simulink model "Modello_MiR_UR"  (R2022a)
settings: Solver=FixedStepAuto  StartTime=0.0  StopTime=time_s(end,1)  FixedStep=Sim.dt*10  RelTol=1e-3  EnableMultiTasking=on
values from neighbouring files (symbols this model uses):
  a = 0.250    (= 0.25)    [Modello_MiR_UR_script.m]    (also in Modello_MiR_2ruote_script.m; Modello_MiR_6ruote_script.m; Modello_MiR_6ruote_validato_script.m)
  a1 = 0.18265    [Modello_MiR_UR_script.m]    (also in UR_DHtable_e.m = 0; Modello_MiR_2ruote_script.m = deg2rad(5); Modello_MiR_6ruote_script.m = deg2rad(5); Modello_MiR_6ruote_validato_script.m)
  a2 = 0.40857    [Modello_MiR_UR_script.m]    (also in UR_DHtable_e.m = 612; Modello_MiR_2ruote_script.m = deg2rad(25); Modello_MiR_6ruote_script.m = deg2rad(25); Modello_MiR_6ruote_validato_script.m)
  Att_C1 = 0.01    [Modello_MiR_UR_script.m]    (also in Modello_MiR_6ruote_validato_script.m)
  Att_C2 = 0.01    [Modello_MiR_UR_script.m]    (also in Modello_MiR_6ruote_validato_script.m)
  Att_C5 = 0.01    [Modello_MiR_UR_script.m]    (also in Modello_MiR_6ruote_validato_script.m)
  Att_C6 = 0.01    [Modello_MiR_UR_script.m]    (also in Modello_MiR_6ruote_validato_script.m)
  b = 0.1875    [Modello_MiR_UR_script.m]    (also in Modello_MiR_2ruote_script.m; Modello_MiR_6ruote_script.m; Modello_MiR_6ruote_validato_script.m)
  b_caster = 0.07    [Modello_MiR_UR_script.m]    (also in Modello_MiR_2ruote_script.m; Modello_MiR_6ruote_script.m; Modello_MiR_6ruote_validato_script.m)
  bd = 0.205    [Modello_MiR_UR_script.m]    (also in Modello_MiR_2ruote_script.m; Modello_MiR_6ruote_script.m; Modello_MiR_6ruote_validato_script.m)
  F23MIR = @(u) (mv*9.801/4)-(mv*h*u(5)+(mv*9.801/4)*(2*a-b_caster*(cos(u(1))+cos(u(2)))))/(4*a-b_caster*(cos(u(1))+cos(u(2)))+b_caster*(cos(u(3))+cos(u(4))))    [Modello_MiR_UR_script.m]
  F23UR5 = @(u) (u(7)/4)-u(11)    [Modello_MiR_UR_script.m]
  F43MIR = @(u) (1/(2*bd))*(mv*u(6)*h+((mv*h*u(5)+(mv*9.801/4)*(2*a-b_caster*(cos(u(1))+cos(u(2)))))/(4*a-b_caster*(cos(u(1))+cos(u(2)))+b_caster*(cos(u(3))+cos(u(4)))))*(2*bd-b_caster*(sin(u(3))+sin(u(4))))+((mv*9.801/4)-(mv*h*u(5)+(mv*9.801/4)*(2*a-b_caster*(cos(u(1))+cos(u(2)))))/(4*a-b_caster*(cos(u(1))+cos(u(2)))+b_caster*(cos(u(3))+cos(u(4)))))*(2*bd-b_caster*(sin(u(1))+sin(u(2)))))    [Modello_MiR_UR_script.m]
  F43UR5 = @(u) (1/(2*bd))*(u(8) - u(6)*H +u(11)*(2*bd-b_caster*(sin(u(3))+sin(u(4))))+u(12)*(2*bd-b_caster*(sin(u(1))+sin(u(2)))))    [Modello_MiR_UR_script.m]
  F63MIR = @(u) (mv*h*u(5)+(mv*9.801/4)*(2*a-b_caster*(cos(u(1))+cos(u(2)))))/(4*a-b_caster*(cos(u(1))+cos(u(2)))+b_caster*(cos(u(3))+cos(u(4))))    [Modello_MiR_UR_script.m]
  F63UR5 = @(u)(-a*u(7)/2 -u(5)*H -u(9) +(u(7)/4)*(2*a-b_caster*(cos(u(1))+cos(u(2)))))/(4*a-b_caster*(cos(u(1))+cos(u(2)))+b_caster*(cos(u(3))+cos(u(4))))    [Modello_MiR_UR_script.m]
  f_c = 0.29564    [Modello_MiR_UR_script.m]    (also in Modello_MiR_6ruote_validato_script.m)
  f_d3 = 0.35846    [Modello_MiR_UR_script.m]    (also in Modello_MiR_6ruote_validato_script.m)
  f_d4 = 0.2333    [Modello_MiR_UR_script.m]    (also in Modello_MiR_6ruote_validato_script.m)
  fa_c = 0.27474    [Modello_MiR_UR_script.m]    (also in Modello_MiR_6ruote_validato_script.m)
  fa_d3 = 0.3694    [Modello_MiR_UR_script.m]    (also in Modello_MiR_6ruote_validato_script.m)
  fa_d4 = 0.28065    [Modello_MiR_UR_script.m]    (also in Modello_MiR_6ruote_validato_script.m)
  fm_fun = @(u) (u <= -am2 || u >= am2) * 0 + (u > -am2 && u <= -am1) * (- u* Mza/(am2 -am1) - Mza* am2/(am2 -am1)) +           + (u > -am1 && u <= am1) * (Mza * u / am1) + (u > am1 && u < am2) * (Mza * u /(am1 -am2) - Mza * am2 /(am1 - am2))    [Modello_MiR_UR_script.m]    (also in Modello_MiR_6ruote_script.m = @(u) (u <= -am2 | u >= am2)*0 + (u > -am2 && u <= -am1)*(- u; Modello_MiR_6ruote_validato_script.m)
  Hi = 1    [UR5e_data.m]
  Icw_1 = 1/2 * mcw * rc^2    (= 0.002004225735)    [Modello_MiR_UR_script.m]    (also in Modello_MiR_2ruote_script.m; Modello_MiR_6ruote_script.m; Modello_MiR_6ruote_validato_script.m)
  Icw_2 = 1/12 * mcw * ec^2 + 1/4 * mcw * rc^2    (= 0.00104098243873)    [Modello_MiR_UR_script.m]    (also in Modello_MiR_2ruote_script.m; Modello_MiR_6ruote_script.m; Modello_MiR_6ruote_validato_script.m)
  Idw_1 = 1/2 * mdw * rd^2    (= 0.00551836278784)    [Modello_MiR_UR_script.m]    (also in Modello_MiR_2ruote_script.m; Transfer_Function_Gol_Gcl.m = Inertia_vect(jj,1); Modello_MiR_6ruote_script.m; Modello_MiR_6ruote_validato_script.m)
  iMax = 20.7*1.1    (= 22.77)    [Modello_MiR_UR_script.m]    (also in Modello_MiR_2ruote_script.m; Modello_MiR_6ruote_script.m; Modello_MiR_6ruote_validato_script.m)
  Iv = mv * (l^2 + w^2)  / 12    (= 6.75343333333)    [Modello_MiR_UR_script.m]    (also in Modello_MiR_2ruote_script.m; Modello_MiR_6ruote_script.m; Modello_MiR_6ruote_validato_script.m = 8.95033333333)
  Kc = 0.15    [Modello_MiR_UR_script.m]    (also in Modello_MiR_2ruote_script.m; Modello_MiR_6ruote_script.m; Modello_MiR_6ruote_validato_script.m)
  Ki_i = 1    [Modello_MiR_UR_script.m]    (also in Modello_MiR_2ruote_script.m; Modello_MiR_6ruote_script.m; Modello_MiR_6ruote_validato_script.m)
  Ki_v = 1    [Modello_MiR_UR_script.m]    (also in Modello_MiR_2ruote_script.m; Modello_MiR_6ruote_script.m; Modello_MiR_6ruote_validato_script.m)
  kk = 0.00005    (= 5e-05)    [Modello_MiR_UR_script.m]    (also in Modello_MiR_2ruote_script.m; Modello_MiR_6ruote_script.m; Modello_MiR_6ruote_validato_script.m)
  Kp_i = 5    [Modello_MiR_UR_script.m]    (also in Modello_MiR_2ruote_script.m; Modello_MiR_6ruote_script.m; Modello_MiR_6ruote_validato_script.m)
  Kp_v = 5    [Modello_MiR_UR_script.m]    (also in Modello_MiR_2ruote_script.m; Modello_MiR_6ruote_script.m; Modello_MiR_6ruote_validato_script.m)
  kv = 1.5e-6    (= 1.5e-06)    [Modello_MiR_UR_script.m]    (also in Modello_MiR_2ruote_script.m; Modello_MiR_6ruote_script.m; Modello_MiR_6ruote_validato_script.m)
  L = R * tauE    (= 0.00181134822805)    [Modello_MiR_UR_script.m]    (also in Modello_MiR_2ruote_script.m; Modello_MiR_6ruote_script.m; Modello_MiR_6ruote_validato_script.m)
  mcw = rc^2 * pi * ec * rhopoliu + 1    (= 1.02616357632)    [Modello_MiR_UR_script.m]    (also in Modello_MiR_2ruote_script.m; Modello_MiR_6ruote_script.m; Modello_MiR_6ruote_validato_script.m)
  mv = 83    [Modello_MiR_UR_script.m]    (also in Modello_MiR_2ruote_script.m; Modello_MiR_6ruote_script.m; Modello_MiR_6ruote_validato_script.m = 110)
  Phi1_start = psi_mir(1,1)    [Modello_MiR_UR_script.m]    (also in Modello_MiR_6ruote_validato_script.m)
  Phi2_start = psi_mir(1,1)    [Modello_MiR_UR_script.m]    (also in Modello_MiR_6ruote_validato_script.m)
  Phi5_start = psi_mir(1,1)    [Modello_MiR_UR_script.m]    (also in Modello_MiR_6ruote_validato_script.m)
  Phi6_start = psi_mir(1,1)    [Modello_MiR_UR_script.m]    (also in Modello_MiR_6ruote_validato_script.m)
  Psi_start = psi_mir(1,1)    [Modello_MiR_UR_script.m]    (also in Modello_MiR_6ruote_script.m = 1.57079632679; Modello_MiR_6ruote_validato_script.m)
  q0 = [qset.q1.signals.values(1),qset.q2.signals.values(1),qset.q3.signals.values(1),qset.q4.signals.values(1),qset.q5.signals.values(1),qset.q6.signals.values(1)]    [UR5e_simmot.m]
  R = velMax * TorqueMax / (iMax)^2    (= 1.81134822805)    [Modello_MiR_UR_script.m]    (also in Modello_MiR_2ruote_script.m; Modello_MiR_6ruote_script.m; Modello_MiR_6ruote_validato_script.m)
  rap_rid = 10.167    [Modello_MiR_UR_script.m]    (also in Modello_MiR_2ruote_script.m; Modello_MiR_6ruote_script.m; Modello_MiR_6ruote_validato_script.m)
  rc = 0.125/2    (= 0.0625)    [Modello_MiR_UR_script.m]    (also in Modello_MiR_2ruote_script.m; Modello_MiR_6ruote_script.m; Modello_MiR_6ruote_validato_script.m)
  rd = 0.1    [Modello_MiR_UR_script.m]    (also in Modello_MiR_2ruote_script.m; Modello_MiR_6ruote_script.m; Modello_MiR_6ruote_validato_script.m)
  s = 1i*s    [Transfer_Function_Gol_Gcl.m]
  s1 = 0.18987    [Modello_MiR_UR_script.m]    (also in Modello_MiR_2ruote_script.m = 0.2; Modello_MiR_6ruote_script.m = 0.2; Modello_MiR_6ruote_validato_script.m)
  s2 = 0.99533    [Modello_MiR_UR_script.m]    (also in Modello_MiR_2ruote_script.m = 0.8; Modello_MiR_6ruote_script.m = 0.8; Modello_MiR_6ruote_validato_script.m)
  Sx = spline(x ,fl_fun(x),zx)    [Modello_MiR_6ruote_script.m]
  Sy = spline(x ,ft_fun(x),zy)    [Modello_MiR_6ruote_script.m]
  tau_i = 1/(2000*2*pi)    (= 7.95774715459e-05)    [UR5e_data.m]    (also in Transfer_Function_Gol_Gcl.m = Kp_i/Ki_i)
  VaMax = Kc * velMax    (= 41.2443991527)    [Modello_MiR_UR_script.m]    (also in Modello_MiR_2ruote_script.m; Modello_MiR_6ruote_script.m; Modello_MiR_6ruote_validato_script.m)
  X_start = traj(1,1)    [Modello_MiR_UR_script.m]    (also in Modello_MiR_2ruote_script.m = input('Inserire coordinata x iniziale'); Modello_MiR_6ruote_script.m = input('Inserire coordinata x iniziale'); Modello_MiR_6ruote_validato_script.m)
  Y_start = traj(1,2)    [Modello_MiR_UR_script.m]    (also in Modello_MiR_2ruote_script.m = input('Inserire coordinata y iniziale'); Modello_MiR_6ruote_script.m = input('Inserire coordinata y iniziale'); Modello_MiR_6ruote_validato_script.m)
undefined symbols (not defined in the file or in its folder): deg, Driver1, Driver2, Driver3, Driver4, Driver5, Driver6, Ground, J1, J2, J3, J4, J5, J6, kg, L1, L2, L3, L4, L5, L6, m, Motor, N, X, Y, z, Z
libraries: sm_lib x33, nesl_utility x30, slpidlib x10
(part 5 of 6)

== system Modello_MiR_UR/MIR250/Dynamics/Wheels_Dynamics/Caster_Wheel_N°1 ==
  Sigma1 : Inport
  alpha1 : Inport  Port=2
  F13 : Inport  Port=3
  parametri_cw1 : Inport  Port=4
  Demux : Demux  Outputs=6
  Slip Forces/Torque : Subsystem
  Wheel Dynamics : Subsystem
  F1L : Outport
  F1T : Outport  Port=2
  Thetad_1 : Outport  Port=3
  Phid_1 : Outport  Port=4
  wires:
  Slip Forces/Torque/1(F1L) -> Wheel Dynamics/1(F1L), F1L/1  "F1L"
  alpha1/1 -> Slip Forces/Torque/2(Alpha1)
  Slip Forces/Torque/2(F1T) -> F1T/1
  Wheel Dynamics/2(Phid_1) -> Phid_1/1
  Sigma1/1 -> Slip Forces/Torque/1(Sigma1)
  Slip Forces/Torque/3(M13) -> Wheel Dynamics/2(M13)
  Wheel Dynamics/1(Thetad_1) -> Thetad_1/1
  F13/1 -> Wheel Dynamics/3(F13), Slip Forces/Torque/3(F13)
  Demux/1 -> Slip Forces/Torque/4(fc1)
  Demux/2 -> Slip Forces/Torque/5(fac1)
  Demux/3 -> Slip Forces/Torque/6(s1)
  Demux/6 -> Slip Forces/Torque/9(a2)
  Demux/5 -> Slip Forces/Torque/8(a1)
  Demux/4 -> Slip Forces/Torque/7(s2)
  parametri_cw1/1 -> Demux/1

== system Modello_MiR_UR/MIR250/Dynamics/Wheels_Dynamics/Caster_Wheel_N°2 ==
  Sigma2 : Inport
  alpha2 : Inport  Port=2
  F23 : Inport  Port=3
  parametri : Inport  Port=4
  Demux : Demux  Outputs=6
  Slip Forces/Torque : Subsystem
  Wheel Dynamics : Subsystem
  F2L : Outport
  F2T : Outport  Port=2
  Thetad_2 : Outport  Port=3
  Phid_2 : Outport  Port=4
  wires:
  Slip Forces/Torque/1(F2L) -> Wheel Dynamics/1(F2L), F2L/1
  alpha2/1 -> Slip Forces/Torque/2(Alpha2)
  Slip Forces/Torque/2(F2T) -> F2T/1
  Wheel Dynamics/2(Phid_2) -> Phid_2/1
  Sigma2/1 -> Slip Forces/Torque/1(Sigma2)
  Slip Forces/Torque/3(M23) -> Wheel Dynamics/2(M23)
  Wheel Dynamics/1(Thetad_2) -> Thetad_2/1
  F23/1 -> Slip Forces/Torque/3(F23), Wheel Dynamics/3(F23)
  Demux/1 -> Slip Forces/Torque/4(fc2)
  Demux/2 -> Slip Forces/Torque/5(fac2)
  Demux/3 -> Slip Forces/Torque/6(s1)
  Demux/4 -> Slip Forces/Torque/7(s2)
  Demux/5 -> Slip Forces/Torque/8(a1)
  Demux/6 -> Slip Forces/Torque/9(a2)
  parametri/1 -> Demux/1

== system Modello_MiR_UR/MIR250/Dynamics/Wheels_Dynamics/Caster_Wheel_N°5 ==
  Sigma5 : Inport
  alpha5 : Inport  Port=2
  F53 : Inport  Port=3
  parametri : Inport  Port=4
  Demux : Demux  Outputs=6
  Slip Forces/Torque : Subsystem
  Wheel Dynamics : Subsystem
  F5L : Outport
  F5T : Outport  Port=2
  Thetad_5 : Outport  Port=3
  Phid_5 : Outport  Port=4
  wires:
  alpha5/1 -> Slip Forces/Torque/2(Alpha5)
  Slip Forces/Torque/2(F5T) -> F5T/1
  Wheel Dynamics/2(Phid_5) -> Phid_5/1
  Sigma5/1 -> Slip Forces/Torque/1(Sigma5)
  Slip Forces/Torque/3(M53) -> Wheel Dynamics/2(M53)
  Wheel Dynamics/1(Thetad_5) -> Thetad_5/1
  F53/1 -> Slip Forces/Torque/3(F53), Wheel Dynamics/3(F53)
  Slip Forces/Torque/1(F5L) -> Wheel Dynamics/1(F5L), F5L/1
  Demux/6 -> Slip Forces/Torque/9(a2)
  Demux/4 -> Slip Forces/Torque/7(s2)
  Demux/1 -> Slip Forces/Torque/4(fc5)
  Demux/5 -> Slip Forces/Torque/8(a1)
  Demux/2 -> Slip Forces/Torque/5(fac5)
  Demux/3 -> Slip Forces/Torque/6(s1)
  parametri/1 -> Demux/1

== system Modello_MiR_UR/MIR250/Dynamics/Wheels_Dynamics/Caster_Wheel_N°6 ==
  Sigma6 : Inport
  alpha6 : Inport  Port=2
  F63 : Inport  Port=3
  parametri : Inport  Port=4
  Demux : Demux  Outputs=6
  Slip Forces/Torque : Subsystem
  Wheel Dynamics : Subsystem
  F6L : Outport
  F6T : Outport  Port=2
  Thetad_6 : Outport  Port=3
  Phid_6 : Outport  Port=4
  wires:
  Slip Forces/Torque/1(F6L) -> Wheel Dynamics/1(F6L), F6L/1
  alpha6/1 -> Slip Forces/Torque/2(Alpha6)
  Slip Forces/Torque/2(F6T) -> F6T/1
  Wheel Dynamics/2(Phid_6) -> Phid_6/1
  Sigma6/1 -> Slip Forces/Torque/1(Sigma6)
  Slip Forces/Torque/3(M63) -> Wheel Dynamics/2(M63)
  Wheel Dynamics/1(Thetad_6) -> Thetad_6/1
  F63/1 -> Slip Forces/Torque/3(F63), Wheel Dynamics/3(F63)
  Demux/6 -> Slip Forces/Torque/9(a2)
  Demux/4 -> Slip Forces/Torque/7(s2)
  Demux/1 -> Slip Forces/Torque/4(fc6)
  Demux/5 -> Slip Forces/Torque/8(a1)
  Demux/2 -> Slip Forces/Torque/5(fac6)
  Demux/3 -> Slip Forces/Torque/6(s1)
  parametri/1 -> Demux/1

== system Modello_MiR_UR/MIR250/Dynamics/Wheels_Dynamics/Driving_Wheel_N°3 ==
  Cm3 : Inport
  Sigma3 : Inport  Port=2
  alpha3 : Inport  Port=3
  F33 : Inport  Port=4
  parametri_dw3 : Inport  Port=5
  Demux : Demux  Outputs=6
  Scope : Scope
  Scope1 : Scope
  Scope2 : Scope
  Subsystem : Subsystem
  Wheel Dynamics : Subsystem
  F3L : Outport
  F3T : Outport  Port=2
  M33 : Outport  Port=3
  Thetad_3 : Outport  Port=4
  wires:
  Cm3/1 -> Wheel Dynamics/1(Cm3)
  Wheel Dynamics/1(Thetad_3) -> Thetad_3/1
  Sigma3/1 -> Subsystem/1(Sigma3)
  alpha3/1 -> Subsystem/2(alpha3)
  Subsystem/1(F3L) -> Scope/1, F3L/1, Wheel Dynamics/2(F3L)  "F3L"
  Subsystem/2(F3T) -> F3T/1, Scope2/1  "F3T"
  Subsystem/3(M33) -> Scope1/1, M33/1
  F33/1 -> Subsystem/3(F33), Wheel Dynamics/3(F33)
  Demux/6 -> Subsystem/9(a2)
  Demux/4 -> Subsystem/7(s2)
  Demux/1 -> Subsystem/4(f)
  Demux/5 -> Subsystem/8(a1)
  Demux/2 -> Subsystem/5(fa)
  Demux/3 -> Subsystem/6(s1)
  parametri_dw3/1 -> Demux/1

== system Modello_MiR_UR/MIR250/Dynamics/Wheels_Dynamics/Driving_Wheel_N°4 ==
  Cm4 : Inport
  Sigma4 : Inport  Port=2
  alpha4 : Inport  Port=3
  F43 : Inport  Port=4
  parametri_dw4 : Inport  Port=5
  Demux : Demux  Outputs=6
  Scope : Scope
  Scope1 : Scope
  Scope2 : Scope
  Subsystem : Subsystem
  Subsystem1 : Subsystem
  F4L : Outport
  F4T : Outport  Port=2
  M43 : Outport  Port=3
  Thetad_4 : Outport  Port=4
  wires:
  Cm4/1 -> Subsystem/1(Cm4)
  alpha4/1 -> Subsystem1/2(alpha4)
  Sigma4/1 -> Subsystem1/1(Sigma4)
  Subsystem1/1(F4L) -> Subsystem/2(F4L), Scope/1, F4L/1
  Subsystem1/2(F4T) -> Scope1/1, F4T/1
  Subsystem1/3(M43) -> Scope2/1, M43/1
  Subsystem/1(Thetad_4) -> Thetad_4/1
  F43/1 -> Subsystem1/3(F43), Subsystem/3(F43)
  Demux/6 -> Subsystem1/9(a2)
  Demux/4 -> Subsystem1/7(s2)
  Demux/1 -> Subsystem1/4(f)
  Demux/5 -> Subsystem1/8(a1)
  Demux/2 -> Subsystem1/5(fa)
  Demux/3 -> Subsystem1/6(s1)
  parametri_dw4/1 -> Demux/1

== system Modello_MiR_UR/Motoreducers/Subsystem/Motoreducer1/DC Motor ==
  Vset : Inport
  qm,qdm,qddm : Inport  Port=2
  Add : Sum  Inputs=+--
  C&V Friction : Subsystem
  Demux1 : Demux  Outputs=3
  Gain : Gain  Gain=Motor.kv_1
  Gain1 : Gain  Gain=1/Motor.L_123
  Gain2 : Gain  Gain=Motor.kc_1
  Gain3 : Gain  Gain=Motor.R_123
  Gain4 : Gain  Gain=Motor.Im_123
  Integrator : Integrator
  Sum : Sum  Inputs=|+-
  Sum1 : Sum  Inputs=|+-
  Terminator : Terminator
  T : Outport  VectorParamsAs1DForOutWhenUnconnected=off
  i : Outport  Port=2
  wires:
  C&V Friction/1(y) -> Sum1/2
  Demux1/1 -> Terminator/1
  qm,qdm,qddm/1 -> Demux1/1
  Demux1/2 -> C&V Friction/1(u), Gain/1
  Sum1/1 -> Sum/1
  Gain2/1 -> Sum1/1  "Electric Torque"
  Vset/1 -> Add/1
  Sum/1 -> T/1
  Demux1/3 -> Gain4/1
  Gain4/1 -> Sum/2
  Gain3/1 -> Add/3
  Integrator/1 -> i/1, Gain2/1, Gain3/1  "Current"
  Gain1/1 -> Integrator/1
  Add/1 -> Gain1/1
  Gain/1 -> Add/2  "Back EMF"

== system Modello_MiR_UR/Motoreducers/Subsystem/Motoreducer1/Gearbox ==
  T : Inport
  q,qd,qdd : Inport  Port=2
  Demux : Demux  Outputs=3
  Gain : Gain  Gain=Motor.eta*Motor.tau
  Gain1 : Gain  Gain=Motor.tau
  Gain2 : Gain  Gain=Motor.tau
  Gain3 : Gain  Gain=Motor.tau
  Mux : Mux  Inputs=3
  Tu : Outport  VectorParamsAs1DForOutWhenUnconnected=off
  qm,qdm,qddm : Outport  Port=2  VectorParamsAs1DForOutWhenUnconnected=off
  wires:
  Mux/1 -> qm,qdm,qddm/1
  Gain1/1 -> Mux/1
  Gain3/1 -> Mux/3
  Gain2/1 -> Mux/2
  q,qd,qdd/1 -> Demux/1
  Demux/3 -> Gain3/1
  Demux/2 -> Gain2/1
  Demux/1 -> Gain1/1
  Gain/1 -> Tu/1
  T/1 -> Gain/1

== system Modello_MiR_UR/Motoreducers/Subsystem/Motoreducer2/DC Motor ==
  Vset : Inport
  qm,qdm,qddm : Inport  Port=2
  Add : Sum  Inputs=+--
  C&V Friction : Subsystem
  Demux1 : Demux  Outputs=3
  Gain : Gain  Gain=Motor.kv_2
  Gain1 : Gain  Gain=1/Motor.L_123
  Gain2 : Gain  Gain=Motor.kc_2
  Gain3 : Gain  Gain=Motor.R_123
  Gain4 : Gain  Gain=Motor.Im_123
  Integrator : Integrator
  Sum : Sum  Inputs=|+-
  Sum1 : Sum  Inputs=|+-
  Terminator : Terminator
  T : Outport  VectorParamsAs1DForOutWhenUnconnected=off
  i : Outport  Port=2
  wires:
  Gain/1 -> Add/2  "Back EMF"
  Add/1 -> Gain1/1
  Gain1/1 -> Integrator/1
  Integrator/1 -> i/1, Gain3/1, Gain2/1  "Current"
  Gain3/1 -> Add/3
  Gain4/1 -> Sum/2
  Demux1/3 -> Gain4/1
  Sum/1 -> T/1
  Vset/1 -> Add/1
  Gain2/1 -> Sum1/1  "Electric Torque"
  Sum1/1 -> Sum/1
  Demux1/2 -> C&V Friction/1(u), Gain/1
  qm,qdm,qddm/1 -> Demux1/1
  Demux1/1 -> Terminator/1
  C&V Friction/1(y) -> Sum1/2

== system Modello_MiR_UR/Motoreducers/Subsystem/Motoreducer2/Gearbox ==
  T : Inport
  q,qd,qdd : Inport  Port=2
  Demux : Demux  Outputs=3
  Gain : Gain  Gain=Motor.eta*Motor.tau
  Gain1 : Gain  Gain=Motor.tau
  Gain2 : Gain  Gain=Motor.tau
  Gain3 : Gain  Gain=Motor.tau
  Mux : Mux  Inputs=3
  Tu : Outport  VectorParamsAs1DForOutWhenUnconnected=off
  qm,qdm,qddm : Outport  Port=2  VectorParamsAs1DForOutWhenUnconnected=off
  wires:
  T/1 -> Gain/1
  Gain/1 -> Tu/1
  Demux/1 -> Gain1/1
  Demux/2 -> Gain2/1
  Demux/3 -> Gain3/1
  q,qd,qdd/1 -> Demux/1
  Gain2/1 -> Mux/2
  Gain3/1 -> Mux/3
  Gain1/1 -> Mux/1
  Mux/1 -> qm,qdm,qddm/1

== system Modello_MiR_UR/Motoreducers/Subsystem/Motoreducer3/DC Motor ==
  Vset : Inport
  qm,qdm,qddm : Inport  Port=2
  Add : Sum  Inputs=+--
  C&V Friction : Subsystem
  Demux1 : Demux  Outputs=3
  Gain : Gain  Gain=Motor.kv_3
  Gain1 : Gain  Gain=1/Motor.L_123
  Gain2 : Gain  Gain=Motor.kc_3
  Gain3 : Gain  Gain=Motor.R_123
  Gain4 : Gain  Gain=Motor.Im_123
  Integrator : Integrator
  Sum : Sum  Inputs=|+-
  Sum1 : Sum  Inputs=|+-
  Terminator : Terminator
  T : Outport  VectorParamsAs1DForOutWhenUnconnected=off
  i : Outport  Port=2
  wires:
  C&V Friction/1(y) -> Sum1/2
  Demux1/1 -> Terminator/1
  qm,qdm,qddm/1 -> Demux1/1
  Demux1/2 -> C&V Friction/1(u), Gain/1
  Sum1/1 -> Sum/1
  Gain2/1 -> Sum1/1  "Electric Torque"
  Vset/1 -> Add/1
  Sum/1 -> T/1
  Demux1/3 -> Gain4/1
  Gain4/1 -> Sum/2
  Gain3/1 -> Add/3
  Integrator/1 -> i/1, Gain2/1, Gain3/1  "Current"
  Gain1/1 -> Integrator/1
  Add/1 -> Gain1/1
  Gain/1 -> Add/2  "Back EMF"

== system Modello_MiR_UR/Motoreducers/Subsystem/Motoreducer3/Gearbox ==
  T : Inport
  q,qd,qdd : Inport  Port=2
  Demux : Demux  Outputs=3
  Gain : Gain  Gain=Motor.eta*Motor.tau
  Gain1 : Gain  Gain=Motor.tau
  Gain2 : Gain  Gain=Motor.tau
  Gain3 : Gain  Gain=Motor.tau
  Mux : Mux  Inputs=3
  Tu : Outport  VectorParamsAs1DForOutWhenUnconnected=off
  qm,qdm,qddm : Outport  Port=2  VectorParamsAs1DForOutWhenUnconnected=off
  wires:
  Mux/1 -> qm,qdm,qddm/1
  Gain1/1 -> Mux/1
  Gain3/1 -> Mux/3
  Gain2/1 -> Mux/2
  q,qd,qdd/1 -> Demux/1
  Demux/3 -> Gain3/1
  Demux/2 -> Gain2/1
  Demux/1 -> Gain1/1
  Gain/1 -> Tu/1
  T/1 -> Gain/1

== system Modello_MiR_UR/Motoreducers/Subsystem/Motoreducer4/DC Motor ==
  Vset : Inport
  qm,qdm,qddm : Inport  Port=2
  Add : Sum  Inputs=+--
  C&V Friction : Subsystem
  Demux1 : Demux  Outputs=3
  Gain : Gain  Gain=Motor.kv_4
  Gain1 : Gain  Gain=1/Motor.L_456
  Gain2 : Gain  Gain=Motor.kc_4
  Gain3 : Gain  Gain=Motor.R_456
  Gain4 : Gain  Gain=Motor.Im_456
  Integrator : Integrator
  Sum : Sum  Inputs=|+-
  Sum1 : Sum  Inputs=|+-
  Terminator : Terminator
  T : Outport  VectorParamsAs1DForOutWhenUnconnected=off
  i : Outport  Port=2
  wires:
  Gain/1 -> Add/2  "Back EMF"
  Add/1 -> Gain1/1
  Gain1/1 -> Integrator/1
  Integrator/1 -> i/1, Gain3/1, Gain2/1  "Current"
  Gain3/1 -> Add/3
  Gain4/1 -> Sum/2
  Demux1/3 -> Gain4/1
  Sum/1 -> T/1
  Vset/1 -> Add/1
  Gain2/1 -> Sum1/1  "Electric Torque"
  Sum1/1 -> Sum/1
  Demux1/2 -> C&V Friction/1(u), Gain/1
  qm,qdm,qddm/1 -> Demux1/1
  Demux1/1 -> Terminator/1
  C&V Friction/1(y) -> Sum1/2

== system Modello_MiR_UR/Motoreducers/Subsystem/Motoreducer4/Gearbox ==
  T : Inport
  q,qd,qdd : Inport  Port=2
  Demux : Demux  Outputs=3
  Gain : Gain  Gain=Motor.eta*Motor.tau
  Gain1 : Gain  Gain=Motor.tau
  Gain2 : Gain  Gain=Motor.tau
  Gain3 : Gain  Gain=Motor.tau
  Mux : Mux  Inputs=3
  Tu : Outport  VectorParamsAs1DForOutWhenUnconnected=off
  qm,qdm,qddm : Outport  Port=2  VectorParamsAs1DForOutWhenUnconnected=off
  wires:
  T/1 -> Gain/1
  Gain/1 -> Tu/1
  Demux/1 -> Gain1/1
  Demux/2 -> Gain2/1
  Demux/3 -> Gain3/1
  q,qd,qdd/1 -> Demux/1
  Gain2/1 -> Mux/2
  Gain3/1 -> Mux/3
  Gain1/1 -> Mux/1
  Mux/1 -> qm,qdm,qddm/1

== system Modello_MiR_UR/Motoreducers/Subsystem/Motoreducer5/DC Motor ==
  Vset : Inport
  qm,qdm,qddm : Inport  Port=2
  Add : Sum  Inputs=+--
  C&V Friction : Subsystem
  Demux1 : Demux  Outputs=3
  Gain : Gain  Gain=Motor.kv_5
  Gain1 : Gain  Gain=1/Motor.L_456
  Gain2 : Gain  Gain=Motor.kc_5
  Gain3 : Gain  Gain=Motor.R_456
  Gain4 : Gain  Gain=Motor.Im_456
  Integrator : Integrator
  Sum : Sum  Inputs=|+-
  Sum1 : Sum  Inputs=|+-
  Terminator : Terminator
  T : Outport  VectorParamsAs1DForOutWhenUnconnected=off
  i : Outport  Port=2
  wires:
  C&V Friction/1(y) -> Sum1/2
  Demux1/1 -> Terminator/1
  qm,qdm,qddm/1 -> Demux1/1
  Demux1/2 -> C&V Friction/1(u), Gain/1
  Sum1/1 -> Sum/1
  Gain2/1 -> Sum1/1  "Electric Torque"
  Vset/1 -> Add/1
  Sum/1 -> T/1
  Demux1/3 -> Gain4/1
  Gain4/1 -> Sum/2
  Gain3/1 -> Add/3
  Integrator/1 -> i/1, Gain2/1, Gain3/1  "Current"
  Gain1/1 -> Integrator/1
  Add/1 -> Gain1/1
  Gain/1 -> Add/2  "Back EMF"

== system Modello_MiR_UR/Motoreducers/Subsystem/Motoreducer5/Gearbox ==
  T : Inport
  q,qd,qdd : Inport  Port=2
  Demux : Demux  Outputs=3
  Gain : Gain  Gain=Motor.eta*Motor.tau
  Gain1 : Gain  Gain=Motor.tau
  Gain2 : Gain  Gain=Motor.tau
  Gain3 : Gain  Gain=Motor.tau
  Mux : Mux  Inputs=3
  Tu : Outport  VectorParamsAs1DForOutWhenUnconnected=off
  qm,qdm,qddm : Outport  Port=2  VectorParamsAs1DForOutWhenUnconnected=off
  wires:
  Mux/1 -> qm,qdm,qddm/1
  Gain1/1 -> Mux/1
  Gain3/1 -> Mux/3
  Gain2/1 -> Mux/2
  q,qd,qdd/1 -> Demux/1
  Demux/3 -> Gain3/1
  Demux/2 -> Gain2/1
  Demux/1 -> Gain1/1
  Gain/1 -> Tu/1
  T/1 -> Gain/1

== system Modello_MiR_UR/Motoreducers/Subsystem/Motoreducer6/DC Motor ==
  Vset : Inport
  qm,qdm,qddm : Inport  Port=2
  Add : Sum  Inputs=+--
  C&V Friction : Subsystem
  Demux1 : Demux  Outputs=3
  Gain : Gain  Gain=Motor.kv_6
  Gain1 : Gain  Gain=1/Motor.L_456
  Gain2 : Gain  Gain=Motor.kc_6
  Gain3 : Gain  Gain=Motor.R_456
  Gain4 : Gain  Gain=Motor.Im_456
  Integrator : Integrator
  Sum : Sum  Inputs=|+-
  Sum1 : Sum  Inputs=|+-
  Terminator : Terminator
  T : Outport  VectorParamsAs1DForOutWhenUnconnected=off
  i : Outport  Port=2
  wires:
  Gain/1 -> Add/2  "Back EMF"
  Add/1 -> Gain1/1
  Gain1/1 -> Integrator/1
  Integrator/1 -> i/1, Gain3/1, Gain2/1  "Current"
  Gain3/1 -> Add/3
  Gain4/1 -> Sum/2
  Demux1/3 -> Gain4/1
  Sum/1 -> T/1
  Vset/1 -> Add/1
  Gain2/1 -> Sum1/1  "Electric Torque"
  Sum1/1 -> Sum/1
  Demux1/2 -> C&V Friction/1(u), Gain/1
  qm,qdm,qddm/1 -> Demux1/1
  Demux1/1 -> Terminator/1
  C&V Friction/1(y) -> Sum1/2

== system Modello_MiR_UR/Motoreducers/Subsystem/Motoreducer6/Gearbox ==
  T : Inport
  q,qd,qdd : Inport  Port=2
  Demux : Demux  Outputs=3
  Gain : Gain  Gain=Motor.eta*Motor.tau
  Gain1 : Gain  Gain=Motor.tau
  Gain2 : Gain  Gain=Motor.tau
  Gain3 : Gain  Gain=Motor.tau
  Mux : Mux  Inputs=3
  Tu : Outport  VectorParamsAs1DForOutWhenUnconnected=off
  qm,qdm,qddm : Outport  Port=2  VectorParamsAs1DForOutWhenUnconnected=off
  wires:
  T/1 -> Gain/1
  Gain/1 -> Tu/1
  Demux/1 -> Gain1/1
  Demux/2 -> Gain2/1
  Demux/3 -> Gain3/1
  q,qd,qdd/1 -> Demux/1
  Gain2/1 -> Mux/2
  Gain3/1 -> Mux/3
  Gain1/1 -> Mux/1
  Mux/1 -> qm,qdm,qddm/1

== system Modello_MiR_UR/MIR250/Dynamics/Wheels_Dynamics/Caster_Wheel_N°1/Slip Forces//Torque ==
  Sigma1 : Inport
  Alpha1 : Inport  Port=2
  F13 : Inport  Port=3
  fc1 : Inport  Port=4
  fac1 : Inport  Port=5
  s1 : Inport  Port=6
  s2 : Inport  Port=7
  a1 : Inport  Port=8
  a2 : Inport  Port=9
  1-D Lookup Table : Lookup_n-D  NumberOfTableDimensions=1  BreakpointsForDimension1Source=Input port  BreakpointsForDimension1=z  TableSource=Input port  Table=Sx  InternalRulePriority=Speed  RndMeth=Simplest
  1-D Lookup Table1 : Lookup_n-D  NumberOfTableDimensions=1  BreakpointsForDimension1Source=Input port  BreakpointsForDimension1=z  TableSource=Input port  Table=Sy  InternalRulePriority=Speed  RndMeth=Simplest
  Gain : Gain  Gain=-1
  Interpreted MATLAB Function3 : MATLABFcn  MATLABFcn=u*b_caster
  MATLAB Function : MATLAB Function  TreatAsAtomicUnit=on
  MATLAB Function1 : MATLAB Function  TreatAsAtomicUnit=on
  Product : Product
  Product1 : Product
  Scope : Scope
  Scope1 : Scope
  F1L : Outport
  F1T : Outport  Port=2
  M13 : Outport  Port=3
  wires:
  F13/1 -> Product/2, Product1/2
  Product/1 -> F1L/1, Scope/1  "F1L"
  Product1/1 -> Gain/1
  Alpha1/1 -> 1-D Lookup Table1/1
  Interpreted MATLAB Function3/1 -> M13/1
  Gain/1 -> F1T/1, Scope1/1, Interpreted MATLAB Function3/1
  Sigma1/1 -> 1-D Lookup Table/1
  1-D Lookup Table/1 -> Product/1
  1-D Lookup Table1/1 -> Product1/1
  MATLAB Function/1(Sx) -> 1-D Lookup Table/2
  MATLAB Function/2(z) -> 1-D Lookup Table/3
  fc1/1 -> MATLAB Function1/1(f), MATLAB Function/1(fc1)  "fc1"
  fac1/1 -> MATLAB Function1/2(fa), MATLAB Function/2(fac1)  "fac1"
  s1/1 -> MATLAB Function/3(s1)
  s2/1 -> MATLAB Function/4(s2)
  MATLAB Function1/1(Sy) -> 1-D Lookup Table1/2
  MATLAB Function1/2(z) -> 1-D Lookup Table1/3
  a1/1 -> MATLAB Function1/3(a1)  "a1"
  a2/1 -> MATLAB Function1/4(a2)  "a2"

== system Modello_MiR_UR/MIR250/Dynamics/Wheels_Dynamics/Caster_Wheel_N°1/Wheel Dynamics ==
  F1L : Inport
  M13 : Inport  Port=2
  F13 : Inport  Port=3
  Gain : Gain  Gain=-rc
  Gain1 : Gain  Gain=1/Icw_1
  Gain2 : Gain  Gain=1/(Icw_2+mcw*b_caster^2)
  Gain3 : Gain  Gain=Att_C1
  Integrator : Integrator
  Integrator1 : Integrator
  Interpreted MATLAB Function : MATLABFcn  MATLABFcn=u(2)*(kk*u(1)+kv*u(1)^2)
  Mux : Mux  Inputs=2
  Mux1 : Mux  Inputs=2
  Scope : Scope
  Scope1 : Scope
  Scope2 : Scope
  Sum : Sum  Inputs=+-
  Sum1 : Sum  Inputs=--
  Thetad_1 : Outport
  Phid_1 : Outport  Port=2  PortDimensions=1
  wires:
  Integrator/1 -> Mux/1, Thetad_1/1
  Sum/1 -> Scope/1, Gain1/1
  Gain1/1 -> Integrator/1
  F1L/1 -> Gain/1
  Gain/1 -> Sum/1
  Interpreted MATLAB Function/1 -> Sum/2
  M13/1 -> Sum1/1, Mux1/1  "M13"
  Sum1/1 -> Gain2/1
  Gain2/1 -> Integrator1/1
  Gain3/1 -> Mux1/2, Sum1/2  "Coppia_Attr"
  Mux/1 -> Interpreted MATLAB Function/1
  F13/1 -> Mux/2
  Mux1/1 -> Scope2/1
  Integrator1/1 -> Scope1/1, Phid_1/1, Gain3/1

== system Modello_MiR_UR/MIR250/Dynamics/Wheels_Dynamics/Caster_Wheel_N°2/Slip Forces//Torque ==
  Sigma2 : Inport
  Alpha2 : Inport  Port=2
  F23 : Inport  Port=3
  fc2 : Inport  Port=4
  fac2 : Inport  Port=5
  s1 : Inport  Port=6
  s2 : Inport  Port=7
  a1 : Inport  Port=8
  a2 : Inport  Port=9
  1-D Lookup Table : Lookup_n-D  NumberOfTableDimensions=1  BreakpointsForDimension1Source=Input port  BreakpointsForDimension1=z  TableSource=Input port  Table=Sx  InternalRulePriority=Speed  RndMeth=Simplest
  1-D Lookup Table1 : Lookup_n-D  NumberOfTableDimensions=1  BreakpointsForDimension1Source=Input port  BreakpointsForDimension1=z  TableSource=Input port  Table=Sy  InternalRulePriority=Speed  RndMeth=Simplest
  Gain : Gain  Gain=-1
  Interpreted MATLAB Function3 : MATLABFcn  MATLABFcn=b_caster*u
  MATLAB Function : MATLAB Function  TreatAsAtomicUnit=on
  MATLAB Function1 : MATLAB Function  TreatAsAtomicUnit=on
  Product : Product
  Product1 : Product
  Scope : Scope
  F2L : Outport
  F2T : Outport  Port=2
  M23 : Outport  Port=3
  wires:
  Product1/1 -> Gain/1
  Gain/1 -> Interpreted MATLAB Function3/1, F2T/1
  Sigma2/1 -> 1-D Lookup Table/1
  Alpha2/1 -> 1-D Lookup Table1/1
  Interpreted MATLAB Function3/1 -> M23/1
  Product/1 -> F2L/1, Scope/1  "F1L"
  F23/1 -> Product1/2, Product/2
  1-D Lookup Table1/1 -> Product1/1
  1-D Lookup Table/1 -> Product/1
  s1/1 -> MATLAB Function/3(s1)
  MATLAB Function/2(z) -> 1-D Lookup Table/3
  MATLAB Function/1(Sx) -> 1-D Lookup Table/2
  s2/1 -> MATLAB Function/4(s2)
  a1/1 -> MATLAB Function1/3(a1)
  MATLAB Function1/1(Sy) -> 1-D Lookup Table1/2
  MATLAB Function1/2(z) -> 1-D Lookup Table1/3
  fc2/1 -> MATLAB Function1/1(f), MATLAB Function/1(fc2)
  a2/1 -> MATLAB Function1/4(a2)
  fac2/1 -> MATLAB Function1/2(fa), MATLAB Function/2(fac2)

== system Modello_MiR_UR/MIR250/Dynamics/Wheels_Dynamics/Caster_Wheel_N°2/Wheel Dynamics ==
  F2L : Inport
  M23 : Inport  Port=2
  F23 : Inport  Port=3
  Gain : Gain  Gain=-rc
  Gain1 : Gain  Gain=1/Icw_1
  Gain2 : Gain  Gain=1/(Icw_2+mcw*b_caster^2)
  Gain3 : Gain  Gain=Att_C2
  Integrator : Integrator
  Integrator1 : Integrator
  Interpreted MATLAB Function : MATLABFcn  MATLABFcn=u(2)*(kk*u(1)+kv*u(1)^2)
  Mux : Mux  Inputs=2
  Mux1 : Mux  Inputs=2
  Scope : Scope
  Scope2 : Scope
  Sum : Sum  Inputs=+-
  Sum1 : Sum  Inputs=--
  Thetad_2 : Outport
  Phid_2 : Outport  Port=2  PortDimensions=1
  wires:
  Integrator/1 -> Mux/1, Thetad_2/1
  Sum/1 -> Scope/1, Gain1/1
  Gain1/1 -> Integrator/1
  F2L/1 -> Gain/1
  Gain/1 -> Sum/1
  Interpreted MATLAB Function/1 -> Sum/2
  Sum1/1 -> Gain2/1
  Gain2/1 -> Integrator1/1
  Mux/1 -> Interpreted MATLAB Function/1
  F23/1 -> Mux/2
  Gain3/1 -> Mux1/2, Sum1/2  "Coppia_Attr"
  Mux1/1 -> Scope2/1
  M23/1 -> Sum1/1, Mux1/1  "M23"
  Integrator1/1 -> Gain3/1, Phid_2/1

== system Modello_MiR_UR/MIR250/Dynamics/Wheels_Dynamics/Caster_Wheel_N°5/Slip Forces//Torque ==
  Sigma5 : Inport
  Alpha5 : Inport  Port=2
  F53 : Inport  Port=3
  fc5 : Inport  Port=4
  fac5 : Inport  Port=5
  s1 : Inport  Port=6
  s2 : Inport  Port=7
  a1 : Inport  Port=8
  a2 : Inport  Port=9
  1-D Lookup Table : Lookup_n-D  NumberOfTableDimensions=1  BreakpointsForDimension1Source=Input port  BreakpointsForDimension1=z  TableSource=Input port  Table=Sx  InternalRulePriority=Speed  RndMeth=Simplest
  1-D Lookup Table1 : Lookup_n-D  NumberOfTableDimensions=1  BreakpointsForDimension1Source=Input port  BreakpointsForDimension1=z  TableSource=Input port  Table=Sy  InternalRulePriority=Speed  RndMeth=Simplest
  Gain : Gain  Gain=-1
  Interpreted MATLAB Function3 : MATLABFcn  MATLABFcn=b_caster*u
  MATLAB Function : MATLAB Function  TreatAsAtomicUnit=on
  MATLAB Function1 : MATLAB Function  TreatAsAtomicUnit=on
  Product : Product
  Product1 : Product
  F5L : Outport
  F5T : Outport  Port=2
  M53 : Outport  Port=3
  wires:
  Product1/1 -> Gain/1
  Gain/1 -> Interpreted MATLAB Function3/1, F5T/1
  Interpreted MATLAB Function3/1 -> M53/1
  Product/1 -> F5L/1  "F1L"
  1-D Lookup Table1/1 -> Product1/1
  1-D Lookup Table/1 -> Product/1
  Alpha5/1 -> 1-D Lookup Table1/1
  Sigma5/1 -> 1-D Lookup Table/1
  F53/1 -> Product1/2, Product/2
  s1/1 -> MATLAB Function/3(s1)
  MATLAB Function/2(z) -> 1-D Lookup Table/3
  MATLAB Function/1(Sx) -> 1-D Lookup Table/2
  s2/1 -> MATLAB Function/4(s2)
  a1/1 -> MATLAB Function1/3(a1)
  MATLAB Function1/1(Sy) -> 1-D Lookup Table1/2
  MATLAB Function1/2(z) -> 1-D Lookup Table1/3
  fc5/1 -> MATLAB Function/1(fc5), MATLAB Function1/1(f)
  a2/1 -> MATLAB Function1/4(a2)
  fac5/1 -> MATLAB Function1/2(fa), MATLAB Function/2(fac5)

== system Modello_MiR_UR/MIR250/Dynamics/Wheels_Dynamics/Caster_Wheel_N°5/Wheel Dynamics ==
  F5L : Inport
  M53 : Inport  Port=2
  F53 : Inport  Port=3
  Gain : Gain  Gain=-rc
  Gain1 : Gain  Gain=1/Icw_1
  Gain2 : Gain  Gain=1/(Icw_2+mcw*b_caster^2)
  Gain3 : Gain  Gain=Att_C5
  Integrator : Integrator
  Integrator1 : Integrator
  Interpreted MATLAB Function : MATLABFcn  MATLABFcn=u(2)*(kk*u(1)+kv*u(1)^2)
  Mux : Mux  Inputs=2
  Mux1 : Mux  Inputs=2
  Scope : Scope
  Scope2 : Scope
  Sum : Sum  Inputs=+-
  Sum1 : Sum  Inputs=--
  Thetad_5 : Outport
  Phid_5 : Outport  Port=2  PortDimensions=1
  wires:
  Integrator/1 -> Mux/1, Thetad_5/1
  Sum/1 -> Scope/1, Gain1/1
  Gain1/1 -> Integrator/1
  F5L/1 -> Gain/1
  Gain/1 -> Sum/1
  Interpreted MATLAB Function/1 -> Sum/2
  Sum1/1 -> Gain2/1
  Gain2/1 -> Integrator1/1
  Mux/1 -> Interpreted MATLAB Function/1
  F53/1 -> Mux/2
  Gain3/1 -> Mux1/2, Sum1/2  "Coppia_Attr"
  Mux1/1 -> Scope2/1
  M53/1 -> Sum1/1, Mux1/1  "M53"
  Integrator1/1 -> Gain3/1, Phid_5/1

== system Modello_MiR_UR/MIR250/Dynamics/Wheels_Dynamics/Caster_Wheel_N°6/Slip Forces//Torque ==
  Sigma6 : Inport
  Alpha6 : Inport  Port=2
  F63 : Inport  Port=3
  fc6 : Inport  Port=4
  fac6 : Inport  Port=5
  s1 : Inport  Port=6
  s2 : Inport  Port=7
  a1 : Inport  Port=8
  a2 : Inport  Port=9
  1-D Lookup Table : Lookup_n-D  NumberOfTableDimensions=1  BreakpointsForDimension1Source=Input port  BreakpointsForDimension1=z  TableSource=Input port  Table=Sx  InternalRulePriority=Speed  RndMeth=Simplest
  1-D Lookup Table1 : Lookup_n-D  NumberOfTableDimensions=1  BreakpointsForDimension1Source=Input port  BreakpointsForDimension1=z  TableSource=Input port  Table=Sy  InternalRulePriority=Speed  RndMeth=Simplest
  Gain : Gain  Gain=-1
  Interpreted MATLAB Function1 : MATLABFcn  MATLABFcn=b_caster*u
  MATLAB Function : MATLAB Function  TreatAsAtomicUnit=on
  MATLAB Function1 : MATLAB Function  TreatAsAtomicUnit=on
  Product : Product
  Product1 : Product
  F6L : Outport
  F6T : Outport  Port=2
  M63 : Outport  Port=3
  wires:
  Product1/1 -> Gain/1
  Gain/1 -> Interpreted MATLAB Function1/1, F6T/1
  Interpreted MATLAB Function1/1 -> M63/1
  1-D Lookup Table1/1 -> Product1/1
  1-D Lookup Table/1 -> Product/1
  Product/1 -> F6L/1  "F1L"
  F63/1 -> Product/2, Product1/2
  Alpha6/1 -> 1-D Lookup Table1/1
  Sigma6/1 -> 1-D Lookup Table/1
  s1/1 -> MATLAB Function/3(s1)
  MATLAB Function/2(z) -> 1-D Lookup Table/3
  MATLAB Function/1(Sx) -> 1-D Lookup Table/2
  s2/1 -> MATLAB Function/4(s2)
  a1/1 -> MATLAB Function1/3(a1)
  MATLAB Function1/1(Sy) -> 1-D Lookup Table1/2
  MATLAB Function1/2(z) -> 1-D Lookup Table1/3
  fc6/1 -> MATLAB Function1/1(f), MATLAB Function/1(fc6)
  a2/1 -> MATLAB Function1/4(a2)
  fac6/1 -> MATLAB Function1/2(fa), MATLAB Function/2(fac6)

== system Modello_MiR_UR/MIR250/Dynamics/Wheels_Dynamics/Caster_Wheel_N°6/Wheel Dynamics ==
  F6L : Inport
  M63 : Inport  Port=2
  F63 : Inport  Port=3
  Gain : Gain  Gain=-rc
  Gain1 : Gain  Gain=1/Icw_1
  Gain2 : Gain  Gain=1/(Icw_2+mcw*b_caster^2)
  Gain3 : Gain  Gain=Att_C6
  Integrator : Integrator
  Integrator1 : Integrator
  Interpreted MATLAB Function : MATLABFcn  MATLABFcn=u(2)*(kk*u(1)+kv*u(1)^2)
  Mux : Mux  Inputs=2
  Mux1 : Mux  Inputs=2
  Scope : Scope
  Scope2 : Scope
  Sum : Sum  Inputs=+-
  Sum1 : Sum  Inputs=--
  Thetad_6 : Outport
  Phid_6 : Outport  Port=2  PortDimensions=1
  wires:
  Integrator/1 -> Mux/1, Thetad_6/1
  Sum/1 -> Scope/1, Gain1/1
  Gain1/1 -> Integrator/1
  F6L/1 -> Gain/1
  Gain/1 -> Sum/1
  Interpreted MATLAB Function/1 -> Sum/2
  Sum1/1 -> Gain2/1
  Gain2/1 -> Integrator1/1
  Mux/1 -> Interpreted MATLAB Function/1
  F63/1 -> Mux/2
  Gain3/1 -> Mux1/2, Sum1/2  "Coppia_Attr"
  Mux1/1 -> Scope2/1
  M63/1 -> Sum1/1, Mux1/1  "M63"
  Integrator1/1 -> Gain3/1, Phid_6/1

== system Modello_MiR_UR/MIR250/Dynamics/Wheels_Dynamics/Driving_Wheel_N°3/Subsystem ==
  Sigma3 : Inport
  alpha3 : Inport  Port=2
  F33 : Inport  Port=3
  f : Inport  Port=4
  fa : Inport  Port=5
  s1 : Inport  Port=6
  s2 : Inport  Port=7
  a1 : Inport  Port=8
  a2 : Inport  Port=9
  1-D Lookup Table : Lookup_n-D  NumberOfTableDimensions=1  BreakpointsForDimension1Source=Input port  BreakpointsForDimension1=z  TableSource=Input port  Table=Sx  InternalRulePriority=Speed  RndMeth=Simplest
  1-D Lookup Table1 : Lookup_n-D  NumberOfTableDimensions=1  BreakpointsForDimension1Source=Input port  BreakpointsForDimension1=z  TableSource=Input port  Table=Sy  InternalRulePriority=Speed  RndMeth=Simplest
  Gain : Gain  Gain=-1
  Gain1 : Gain  Gain=0.3
  Interpreted MATLAB Function1 : MATLABFcn  MATLABFcn=fm_fun(u)
  MATLAB Function : MATLAB Function  TreatAsAtomicUnit=on
  MATLAB Function1 : MATLAB Function  TreatAsAtomicUnit=on
  Product : Product
  Product1 : Product
  Product2 : Product
  F3L : Outport
  F3T : Outport  Port=2
  M33 : Outport  Port=3
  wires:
  Gain/1 -> F3T/1
  Interpreted MATLAB Function1/1 -> Gain1/1
  F33/1 -> Product2/2, Product1/2, Product/2
  alpha3/1 -> Interpreted MATLAB Function1/1, 1-D Lookup Table1/1
  Product1/1 -> Gain/1
  Product/1 -> F3L/1  "F1L"
  1-D Lookup Table1/1 -> Product1/1
  1-D Lookup Table/1 -> Product/1
  Sigma3/1 -> 1-D Lookup Table/1
  s1/1 -> MATLAB Function/3(s1)
  MATLAB Function/2(z) -> 1-D Lookup Table/3
  MATLAB Function/1(Sx) -> 1-D Lookup Table/2
  s2/1 -> MATLAB Function/4(s2)
  a1/1 -> MATLAB Function1/3(a1)
  MATLAB Function1/1(Sy) -> 1-D Lookup Table1/2
  MATLAB Function1/2(z) -> 1-D Lookup Table1/3
  f/1 -> MATLAB Function1/1(f), MATLAB Function/1(f)
  a2/1 -> MATLAB Function1/4(a2)
  fa/1 -> MATLAB Function1/2(fa), MATLAB Function/2(fa)
  Product2/1 -> M33/1
  Gain1/1 -> Product2/1

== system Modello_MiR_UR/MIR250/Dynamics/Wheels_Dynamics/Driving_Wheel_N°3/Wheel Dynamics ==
  Cm3 : Inport
  F3L : Inport  Port=2
  F33 : Inport  Port=3
  Gain : Gain  Gain=rd
  Gain1 : Gain  Gain=1/(Idw_1+2*10^(-3))
  Integrator : Integrator
  Interpreted MATLAB Function : MATLABFcn  MATLABFcn=u(2)*(kk*u(1)+kv*u(1)^2)
  Mux : Mux  Inputs=2
  Scope : Scope
  Sum : Sum  Inputs=+--
  Thetad_3 : Outport
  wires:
  Cm3/1 -> Sum/1
  Gain/1 -> Sum/2
  Interpreted MATLAB Function/1 -> Sum/3
  Integrator/1 -> Mux/1, Thetad_3/1
  Sum/1 -> Scope/1, Gain1/1
  Gain1/1 -> Integrator/1
  F3L/1 -> Gain/1
  Mux/1 -> Interpreted MATLAB Function/1
  F33/1 -> Mux/2

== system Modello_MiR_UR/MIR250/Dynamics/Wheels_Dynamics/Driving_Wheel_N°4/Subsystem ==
  Cm4 : Inport
  F4L : Inport  Port=2
  F43 : Inport  Port=3
  Gain : Gain  Gain=rd
  Gain1 : Gain  Gain=1/(Idw_1+2*10^(-3))
  Integrator : Integrator
  Interpreted MATLAB Function : MATLABFcn  MATLABFcn=u(2)*(kk*u(1)+kv*u(1)^2)
  Mux : Mux  Inputs=3
  Mux1 : Mux  Inputs=2
  Scope : Scope
  Sum : Sum  Inputs=+--
  Thetad_4 : Outport
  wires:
  Interpreted MATLAB Function/1 -> Mux/2, Sum/3  "Res_rot"
  Gain/1 -> Mux/3, Sum/2  "rd*Fc_R"
  Sum/1 -> Gain1/1
  Gain1/1 -> Integrator/1
  Integrator/1 -> Mux1/1, Thetad_4/1
  F4L/1 -> Gain/1
  Cm4/1 -> Mux/1, Sum/1  "Cm_R"
  Mux/1 -> Scope/1
  Mux1/1 -> Interpreted MATLAB Function/1
  F43/1 -> Mux1/2

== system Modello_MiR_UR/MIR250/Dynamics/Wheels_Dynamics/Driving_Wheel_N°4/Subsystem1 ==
  Sigma4 : Inport
  alpha4 : Inport  Port=2
  F43 : Inport  Port=3
  f : Inport  Port=4
  fa : Inport  Port=5
  s1 : Inport  Port=6
  s2 : Inport  Port=7
  a1 : Inport  Port=8
  a2 : Inport  Port=9
  1-D Lookup Table : Lookup_n-D  NumberOfTableDimensions=1  BreakpointsForDimension1Source=Input port  BreakpointsForDimension1=z  TableSource=Input port  Table=Sx  InternalRulePriority=Speed  RndMeth=Simplest
  1-D Lookup Table1 : Lookup_n-D  NumberOfTableDimensions=1  BreakpointsForDimension1Source=Input port  BreakpointsForDimension1=z  TableSource=Input port  Table=Sy  InternalRulePriority=Speed  RndMeth=Simplest
  Gain : Gain  Gain=-1
  Gain1 : Gain  Gain=0.3
  Interpreted MATLAB Function1 : MATLABFcn  MATLABFcn=fm_fun(u)
  MATLAB Function : MATLAB Function  TreatAsAtomicUnit=on
  MATLAB Function1 : MATLAB Function  TreatAsAtomicUnit=on
  Product : Product
  Product1 : Product
  Product2 : Product
  F4L : Outport
  F4T : Outport  Port=2
  M43 : Outport  Port=3
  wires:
  Gain/1 -> F4T/1
  Interpreted MATLAB Function1/1 -> Gain1/1
  F43/1 -> Product2/2, Product/2, Product1/2
  alpha4/1 -> Interpreted MATLAB Function1/1, 1-D Lookup Table1/1
  Product1/1 -> Gain/1
  Product/1 -> F4L/1  "F1L"
  1-D Lookup Table1/1 -> Product1/1
  1-D Lookup Table/1 -> Product/1
  Sigma4/1 -> 1-D Lookup Table/1
  s1/1 -> MATLAB Function/3(s1)
  MATLAB Function/2(z) -> 1-D Lookup Table/3
  MATLAB Function/1(Sx) -> 1-D Lookup Table/2
  s2/1 -> MATLAB Function/4(s2)
  a1/1 -> MATLAB Function1/3(a1)
  MATLAB Function1/1(Sy) -> 1-D Lookup Table1/2
  MATLAB Function1/2(z) -> 1-D Lookup Table1/3
  f/1 -> MATLAB Function1/1(f), MATLAB Function/1(f)
  a2/1 -> MATLAB Function1/4(a2)
  fa/1 -> MATLAB Function1/2(fa), MATLAB Function/2(fa)
  Gain1/1 -> Product2/1
  Product2/1 -> M43/1

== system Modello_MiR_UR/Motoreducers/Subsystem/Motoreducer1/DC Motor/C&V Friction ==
  u : Inport
  Constant : Constant  Value=J1.Cp
  Constant1 : Constant  Value=J1.Cn
  Gain : Gain  Gain=J1.B
  Sign : Signum
  Sum : Sum  Inputs=|++
  Switch : Switch
  y : Outport
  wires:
  u/1 -> Sign/1, Gain/1
  Sign/1 -> Switch/2
  Constant/1 -> Switch/1
  Constant1/1 -> Switch/3
  Switch/1 -> Sum/2
  Gain/1 -> Sum/1
  Sum/1 -> y/1

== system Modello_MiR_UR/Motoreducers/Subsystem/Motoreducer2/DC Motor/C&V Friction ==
  u : Inport
  Constant : Constant  Value=J2.Cp
  Constant1 : Constant  Value=J2.Cn
  Gain : Gain  Gain=J2.B
  Sign : Signum
  Sum : Sum  Inputs=|++
  Switch : Switch
  y : Outport
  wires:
  u/1 -> Sign/1, Gain/1
  Sign/1 -> Switch/2
  Constant/1 -> Switch/1
  Constant1/1 -> Switch/3
  Switch/1 -> Sum/2
  Gain/1 -> Sum/1
  Sum/1 -> y/1

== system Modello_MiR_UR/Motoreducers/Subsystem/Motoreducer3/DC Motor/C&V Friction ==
  u : Inport
  Constant : Constant  Value=J3.Cp
  Constant1 : Constant  Value=J3.Cn
  Gain : Gain  Gain=J3.B
  Sign : Signum
  Sum : Sum  Inputs=|++
  Switch : Switch
  y : Outport
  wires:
  u/1 -> Sign/1, Gain/1
  Sign/1 -> Switch/2
  Constant/1 -> Switch/1
  Constant1/1 -> Switch/3
  Switch/1 -> Sum/2
  Gain/1 -> Sum/1
  Sum/1 -> y/1

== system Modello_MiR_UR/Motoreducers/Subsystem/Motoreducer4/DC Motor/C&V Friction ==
  u : Inport
  Constant : Constant  Value=J3.Cp
  Constant1 : Constant  Value=J3.Cn
  Gain : Gain  Gain=J3.B
  Sign : Signum
  Sum : Sum  Inputs=|++
  Switch : Switch
  y : Outport
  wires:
  u/1 -> Sign/1, Gain/1
  Sign/1 -> Switch/2
  Constant/1 -> Switch/1
  Constant1/1 -> Switch/3
  Switch/1 -> Sum/2
  Gain/1 -> Sum/1
  Sum/1 -> y/1

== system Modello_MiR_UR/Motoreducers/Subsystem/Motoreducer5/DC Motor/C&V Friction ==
  u : Inport
  Constant : Constant  Value=J5.Cp
  Constant1 : Constant  Value=J5.Cn
  Gain : Gain  Gain=J5.B
  Sign : Signum
  Sum : Sum  Inputs=|++
  Switch : Switch
  y : Outport
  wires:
  u/1 -> Sign/1, Gain/1
  Sign/1 -> Switch/2
  Constant/1 -> Switch/1
  Constant1/1 -> Switch/3
  Switch/1 -> Sum/2
  Gain/1 -> Sum/1
  Sum/1 -> y/1

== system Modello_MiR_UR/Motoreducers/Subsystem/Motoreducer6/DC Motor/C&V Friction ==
  u : Inport
  Constant : Constant  Value=J6.Cp
  Constant1 : Constant  Value=J6.Cn
  Gain : Gain  Gain=J6.B
  Sign : Signum
  Sum : Sum  Inputs=|++
  Switch : Switch
  y : Outport
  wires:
  u/1 -> Sign/1, Gain/1
  Sign/1 -> Switch/2
  Constant/1 -> Switch/1
  Constant1/1 -> Switch/3
  Switch/1 -> Sum/2
  Gain/1 -> Sum/1
  Sum/1 -> y/1

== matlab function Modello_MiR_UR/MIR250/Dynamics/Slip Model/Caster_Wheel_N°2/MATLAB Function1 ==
function Fc_pos_out = fcn(v_wheel,Vx_DL)
x=v_wheel;
y=Vx_DL;
cccc=1e20;

Fc_pos=@(x,y) ((((x-y)/abs(x+((1/cccc)*(x==0))))*(((x-y)/abs(x+((1/cccc)*(x==0))))<=1 )+ 1*(((x-y)/abs(x+((1/cccc)*(x==0))))>1))*(x*y>=0 && x>=0) + (((x-y)/abs(y+((1/cccc)*(y==0))))*(((x-y)/abs(y+((1/cccc)*(y==0))))<=1 ))*(x*y>0 && x<0)+ (x*y<0)*(x/abs(x+((1/cccc)*(x==0)))))*(0.02<(x^2+y^2)) + (10*(x-y)*(10*(x-y)<1) +1*(10*(x-y)>=1))*(0.02>=(x^2+y^2));

Fc_pos_out = Fc_pos(x,y);

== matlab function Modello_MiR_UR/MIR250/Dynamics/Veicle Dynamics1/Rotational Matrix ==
function [Fx_generalized, Fy_generalized] = fcn(FL,FT,Delta)
Fx_generalized=ones(6,1);
Fy_generalized=ones(6,1);

Fx_generalized(1,1)=FL(1)*cos(Delta(1))-FT(1)*sin(Delta(1));
Fy_generalized(1,1)=FT(1)*cos(Delta(1))+FL(1)*sin(Delta(1));
Fx_generalized(2,1)=FL(2)*cos(Delta(2))-FT(2)*sin(Delta(2));
Fy_generalized(2,1)=FT(2)*cos(Delta(2))+FL(2)*sin(Delta(2));
Fx_generalized(3,1)=FL(3);
Fy_generalized(3,1)=FT(3);
Fx_generalized(4,1)=FL(4);
Fy_generalized(4,1)=FT(4);
Fx_generalized(5,1)=FL(5)*cos(Delta(3))-FT(5)*sin(Delta(3));
Fy_generalized(5,1)=FT(5)*cos(Delta(3))+FL(5)*sin(Delta(3));
Fx_generalized(6,1)=FL(6)*cos(Delta(4))-FT(6)*sin(Delta(4));
Fy_generalized(6,1)=FT(6)*cos(Delta(4))+FL(6)*sin(Delta(4));

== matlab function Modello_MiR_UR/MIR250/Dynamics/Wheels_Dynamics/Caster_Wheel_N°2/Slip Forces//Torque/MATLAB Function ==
function [Sx, z] = fcn(fc2, fac2, s1, s2)
f=fc2;
fa=fac2;
FLa =  fa  ;
FL = f  ;
Fx = @(u) (u <= -s2).* (-FL) + (u > -s2 & u <= -s1).*(u*(FL - FLa)/(s2 - s1) + s2*(FL - FLa)/(s2 - s1) - FL) +...
        + (u > -s1 & u <= s1).*(u * FLa / s1) + (u > s1 & u <= s2).* (u * (FLa - FL)/(s1 - s2) - s2 * (FLa - FL)/(s1 - s2) + FL) + ...
        + (u> s2) * FL;
% Interpolazione Cubica Attrito Longitudinale
nvet = 23 ; %specificare i numeri di nodi ( −1) della partizione
inferior = -1; % estremo inferiore intervallo
superi = 1 ; % estremo superiore intervallo
z = linspace(inferior,superi,10001); % definisco la griglia fine su cui valutare la spline
%figure
%set(gcf,'Position',[381 175 1208 753])

n = nvet ;
x = linspace(inferior, superi, n+1); % in questo esercizio definisco i nodi di interpolazione tra loro equispaziati
Sx = spline(x ,Fx(x),z) ; % valuto la spline cubica interpolante

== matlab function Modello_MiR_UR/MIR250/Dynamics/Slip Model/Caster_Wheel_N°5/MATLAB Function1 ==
function Fc_pos_out = fcn(v_wheel,Vx_DL)
x=v_wheel;
y=Vx_DL;
cccc=1e20;

Fc_pos=@(x,y) ((((x-y)/abs(x+((1/cccc)*(x==0))))*(((x-y)/abs(x+((1/cccc)*(x==0))))<=1 )+ 1*(((x-y)/abs(x+((1/cccc)*(x==0))))>1))*(x*y>=0 && x>=0) + (((x-y)/abs(y+((1/cccc)*(y==0))))*(((x-y)/abs(y+((1/cccc)*(y==0))))<=1 ))*(x*y>0 && x<0)+ (x*y<0)*(x/abs(x+((1/cccc)*(x==0)))))*(0.02<(x^2+y^2)) + (10*(x-y)*(10*(x-y)<1) +1*(10*(x-y)>=1))*(0.02>=(x^2+y^2));

Fc_pos_out = Fc_pos(x,y);

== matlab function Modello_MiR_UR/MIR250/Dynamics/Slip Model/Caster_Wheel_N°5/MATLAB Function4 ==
function Fc_neg_out = fcn(v_wheel,Vx_DL)
x=v_wheel;
y=Vx_DL;
cccc=1e20;

Fc_neg=@(x,y) ((((x-y)/abs(y+((1/cccc)*(y==0))))*(((x-y)/abs(y+((1/cccc)*(y==0))))>=-1)+ (-1)*(((x-y)/abs(y+((1/cccc)*(y==0))))<-1))*(x*y>=0 && y>=0) + (((x-y)/abs(x+((1/cccc)*(x==0))))*(((x-y)/abs(x+((1/cccc)*(x==0))))>=-1))*(x*y>0 && y<0) + (x*y<0)*(x/abs(x+((1/cccc)*(x==0)))) )*(0.02<(x^2+y^2)) +(10*(x-y)*(10*(x-y)>-1) -1*(10*(x-y)<=-1))*(0.02>=(x^2+y^2)); 
Fc_neg_out = Fc_neg(x,y);

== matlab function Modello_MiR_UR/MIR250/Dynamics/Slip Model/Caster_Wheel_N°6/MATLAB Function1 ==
function Fc_pos_out = fcn(v_wheel,Vx_DL)

x=v_wheel;
y=Vx_DL;
cccc=1e20;

Fc_pos=@(x,y) ((((x-y)/abs(x+((1/cccc)*(x==0))))*(((x-y)/abs(x+((1/cccc)*(x==0))))<=1 )+ 1*(((x-y)/abs(x+((1/cccc)*(x==0))))>1))*(x*y>=0 && x>=0) + (((x-y)/abs(y+((1/cccc)*(y==0))))*(((x-y)/abs(y+((1/cccc)*(y==0))))<=1 ))*(x*y>0 && x<0)+ (x*y<0)*(x/abs(x+((1/cccc)*(x==0)))))*(0.02<(x^2+y^2)) + (10*(x-y)*(10*(x-y)<1) +1*(10*(x-y)>=1))*(0.02>=(x^2+y^2));

Fc_pos_out = Fc_pos(x,y);

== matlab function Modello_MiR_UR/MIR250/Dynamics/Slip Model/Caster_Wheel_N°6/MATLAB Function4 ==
function Fc_neg_out = fcn(v_wheel,Vx_DL)
x=v_wheel;
y=Vx_DL;
cccc=1e20;

Fc_neg=@(x,y) ((((x-y)/abs(y+((1/cccc)*(y==0))))*(((x-y)/abs(y+((1/cccc)*(y==0))))>=-1)+ (-1)*(((x-y)/abs(y+((1/cccc)*(y==0))))<-1))*(x*y>=0 && y>=0) + (((x-y)/abs(x+((1/cccc)*(x==0))))*(((x-y)/abs(x+((1/cccc)*(x==0))))>=-1))*(x*y>0 && y<0) + (x*y<0)*(x/abs(x+((1/cccc)*(x==0)))) )*(0.02<(x^2+y^2)) +(10*(x-y)*(10*(x-y)>-1) -1*(10*(x-y)<=-1))*(0.02>=(x^2+y^2)); 
Fc_neg_out = Fc_neg(x,y);

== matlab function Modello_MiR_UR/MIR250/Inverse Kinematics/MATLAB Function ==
function Thetad_DR_SET = angvelR( xd_set, psid_set)
 bd = 0.2050;
 rd = 0.1;
Thetad_DR_SET = 1/rd * (xd_set + bd*psid_set);

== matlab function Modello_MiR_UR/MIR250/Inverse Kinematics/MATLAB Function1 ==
function Thetad_DL_SET = angvelL(xd_set,  psid_set)
 bd = 0.2050;
 rd = 0.1;
Thetad_DL_SET = 1/rd * (xd_set - bd*psid_set);

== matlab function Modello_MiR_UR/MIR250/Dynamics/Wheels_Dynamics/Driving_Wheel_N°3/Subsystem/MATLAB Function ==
function [Sx, z] = fcn(f, fa, s1, s2)
FLa =  fa  ;
FL = f  ;
Fx = @(u) (u <= -s2).* (-FL) + (u > -s2 & u <= -s1).*(u*(FL - FLa)/(s2 - s1) + s2*(FL - FLa)/(s2 - s1) - FL) +...
        + (u > -s1 & u <= s1).*(u * FLa / s1) + (u > s1 & u <= s2).* (u * (FLa - FL)/(s1 - s2) - s2 * (FLa - FL)/(s1 - s2) + FL) + ...
        + (u> s2) * FL;
% Interpolazione Cubica Attrito Longitudinale
nvet = 23 ; %specificare i numeri di nodi ( −1) della partizione
inferior = -1; % estremo inferiore intervallo
superi = 1 ; % estremo superiore intervallo
z = linspace(inferior,superi,10001); % definisco la griglia fine su cui valutare la spline
%figure
%set(gcf,'Position',[381 175 1208 753])

n = nvet ;
x = linspace(inferior, superi, n+1); % in questo esercizio definisco i nodi di interpolazione tra loro equispaziati
Sx = spline(x ,Fx(x),z) ; % valuto la spline cubica interpolante
